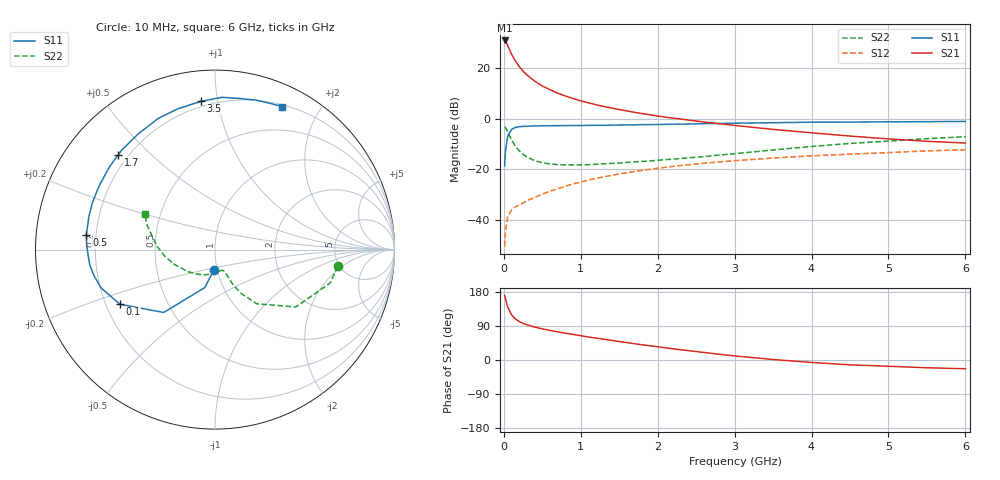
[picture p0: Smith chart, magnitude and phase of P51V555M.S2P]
! SIEMENS Small Signal Semiconductors
! BFP183
! Si NPN RF Bipolar Junction Transistor in SOT143
! VCE = 1.5 V  IC = 55 mA
! Common Emitter S-Parameters:  March  1996
# GHz  S  MA  R  50
!  f  S11  S21  S12  S22
! GHz  MAG  ANG  MAG  ANG  MAG  ANG  MAG  ANG
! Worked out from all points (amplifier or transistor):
!   36 points, 10 MHz to 6 GHz, reference 50 ohm
!   highest |S21| = 30.9 dB at 10 MHz (marker M1)
!   |S21| within 3 dB of that: start of sweep to 65.5 MHz
!   unconditionally stable (mu >= 1): start of sweep to 32.14 MHz; 161.7 MHz to end of sweep
!   at 250 MHz: K = 1.27, MAG = 23.0 dB, |S12| = -33.4 dB
!   at 1.4 GHz: K = 1.81, MAG = 8.1 dB, |S12| = -22.4 dB
!   at 6 GHz: K = 1.43, MAG = -2.6 dB, |S12| = -12.3 dB
!   S11 on the Smith chart (normalised r, x): 10 MHz: 0.96, -0.22; 100 MHz: 0.26, -0.25; 500 MHz: 0.16, +0.06; 1.7 GHz: 0.16, +0.40; 3.5 GHz: 0.17, +0.90; 6 GHz: 0.22, +1.55
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0.01  0.1157 -93.5  35.17 171.0  0.003 61.9  0.6893 -7.8
0.02  0.2188 -105.0  34.2 162.2  0.0058 64.9  0.6689 -16.1
0.05  0.4521 -129.2  28.14 140.2  0.0115 58.9  0.552 -35.4
0.1  0.6111 -150.1  18.96 119.4  0.0156 44.7  0.3815 -52.3
0.15  0.6702 -161.5  13.79 108.4  0.018 44.6  0.2859 -59.1
0.2  0.6902 -168.0  10.7 101.5  0.0196 46.0  0.2306 -62.2
0.25  0.7026 -172.8  8.699 96.6  0.0215 47.6  0.1967 -63.6
0.3  0.7065 -176.5  7.315 93.0  0.0238 49.9  0.1739 -64.2
0.4  0.7156 177.8  5.535 86.9  0.0275 53.3  0.1476 -65.4
0.5  0.7215 173.4  4.428 82.3  0.0321 55.5  0.1341 -66.7
0.6  0.722 169.1  3.734 78.0  0.0368 58.1  0.127 -68.1
0.7  0.7265 165.3  3.187 74.3  0.041 60.0  0.123 -70.0
0.9  0.7312 159.4  2.502 67.5  0.0513 60.3  0.1215 -75.3
1.1  0.7351 152.6  2.051 60.7  0.061 60.3  0.1226 -81.2
1.3  0.7389 147.0  1.733 54.7  0.0706 59.5  0.1276 -87.4
1.7  0.7537 135.6  1.331 42.9  0.0902 56.7  0.1395 -100.7
2.2  0.7744 123.1  1.023 29.5  0.1137 51.7  0.1581 -118.6
2.8  0.8017 109.0  0.795 15.1  0.1392 44.9  0.1904 -138.8
3.5  0.8297 95.4  0.613 1.3  0.1663 37.3  0.24 -159.7
4.5  0.8535 80.4  0.452 -12.9  0.1981 26.3  0.323 176.9
5.5  0.8704 69.5  0.356 -20.5  0.2303 16.6  0.4015 160.3
6  0.8807 64.8  0.329 -23.1  0.2422 11.4  0.4385 153.2
